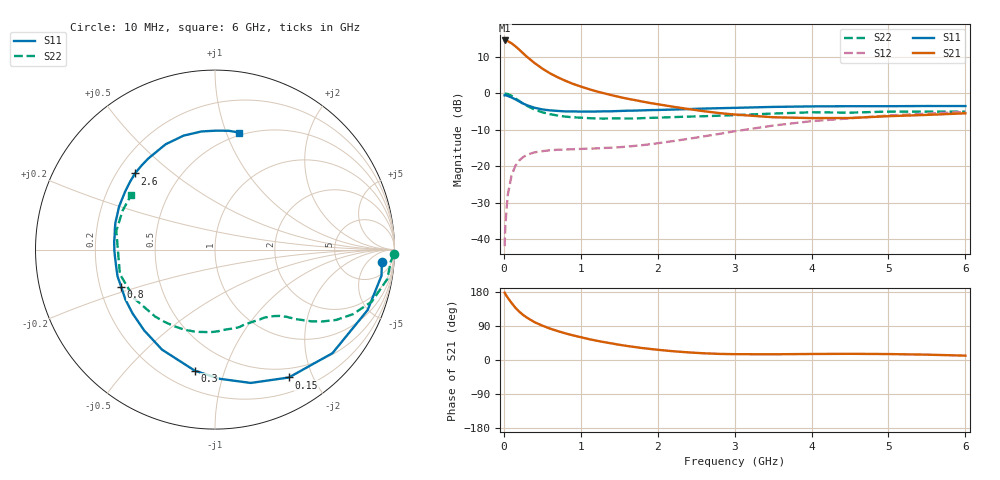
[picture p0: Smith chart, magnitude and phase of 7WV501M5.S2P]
! Infineon Technologies  Discrete & RF Semiconductors
! BFS17W
! Si NPN RF Bipolar Junction Transistor in SOT323
! VCE = 0.5 V  IC = 1.5 mA
! Common Emitter S-Parameters:  August  1999
# GHz  S  MA  R  50
!  f  S11  S21  S12  S22
! GHz  MAG  ANG  MAG  ANG  MAG  ANG  MAG  ANG
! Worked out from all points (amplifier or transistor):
!   36 points, 10 MHz to 6 GHz, reference 50 ohm
!   highest |S21| = 14.4 dB at 10 MHz (marker M1)
!   |S21| within 3 dB of that: start of sweep to 224.7 MHz
!   unconditionally stable (mu >= 1): 780 MHz to end of sweep
!   at 250 MHz: K = 0.36, MSG = 14.2 dB, |S12| = -17.5 dB
!   at 1.4 GHz: K = 1.47, MAG = 3.1 dB, |S12| = -14.9 dB
!   at 6 GHz: K = 1.15, MAG = -2.6 dB, |S12| = -5.1 dB
!   S11 on the Smith chart (normalised r, x): 10 MHz: 14, -14; 150 MHz: 0.38, -1.67; 300 MHz: 0.31, -0.80; 800 MHz: 0.29, -0.18; 2.6 GHz: 0.27, +0.37; 6 GHz: 0.47, +1.11
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0.01  0.932 -4.2  5.245 177.7  0.0081 86.8  0.9966 -1.5
0.02  0.939 -8.9  5.244 173.9  0.0158 89.1  0.9814 -3.9
0.05  0.9147 -21.6  5.147 164.6  0.0401 77.9  0.9741 -9.7
0.1  0.8725 -41.4  4.795 150.7  0.0749 66.3  0.9208 -18.3
0.15  0.8228 -60.0  4.37 138.0  0.1014 56.4  0.8485 -25.1
0.2  0.7691 -75.0  3.928 127.7  0.1203 49.3  0.7812 -30.1
0.25  0.7199 -88.1  3.506 119.0  0.1332 43.1  0.7181 -33.9
0.3  0.6838 -99.5  3.138 111.8  0.1435 39.0  0.6705 -36.6
0.4  0.6307 -117.9  2.577 99.8  0.1553 32.8  0.5953 -40.6
0.5  0.5988 -131.2  2.166 90.7  0.1609 29.2  0.5472 -43.2
0.6  0.5809 -142.2  1.865 82.9  0.1655 27.1  0.5155 -45.8
0.8  0.5623 -158.2  1.475 70.3  0.1694 25.5  0.4776 -51.7
1.1  0.5587 -175.5  1.138 55.4  0.1742 26.4  0.4553 -61.3
1.3  0.5636 175.4  0.997 47.3  0.1781 28.3  0.4489 -68.8
1.6  0.5749 164.7  0.841 37.1  0.1856 32.3  0.4493 -79.9
2.2  0.5962 147.0  0.652 23.1  0.2209 40.5  0.4699 -102.8
2.6  0.6154 136.4  0.566 17.7  0.2565 43.4  0.4836 -117.9
3.5  0.6481 115.1  0.468 15.1  0.3601 41.5  0.5258 -148.8
4  0.6587 105.4  0.456 15.9  0.4139 36.8  0.5472 -165.6
4.5  0.6626 96.5  0.457 16.3  0.4524 31.6  0.541 -179.9
5.5  0.6665 83.4  0.504 14.1  0.5248 22.1  0.5586 157.1
6  0.6658 78.4  0.53 11.5  0.5554 17.2  0.5578 147.0
